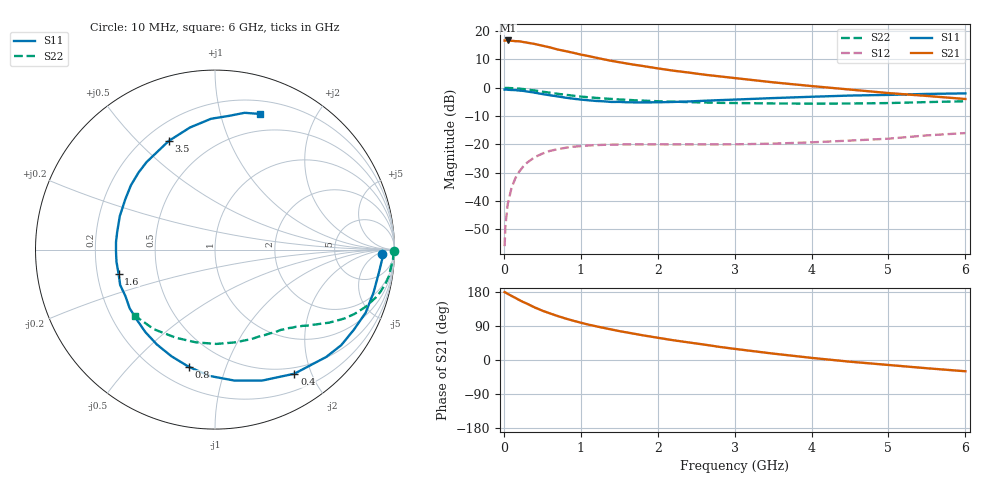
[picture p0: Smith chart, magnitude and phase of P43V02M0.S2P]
! SIEMENS Small Signal Semiconductors
! BFP182
! Si NPN RF Bipolar Junction Transistor in SOT143
! VCE = 3 V  IC = 2 mA
! Common Emitter S-Parameters:  March  1996
# GHz  S  MA  R  50
!  f  S11  S21  S12  S22
! GHz  MAG  ANG  MAG  ANG  MAG  ANG  MAG  ANG
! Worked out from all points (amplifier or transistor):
!   36 points, 10 MHz to 6 GHz, reference 50 ohm
!   highest |S21| = 16.7 dB at 50 MHz (marker M1)
!   |S21| within 3 dB of that: start of sweep to 673.9 MHz
!   unconditionally stable (mu >= 1): 2.189 GHz to 5.892 GHz
!   at 250 MHz: K = 0.13, MSG = 22.0 dB, |S12| = -27.9 dB
!   at 1.4 GHz: K = 0.68, MSG = 14.8 dB, |S12| = -20.1 dB
!   at 6 GHz: K = 0.99, MSG = 6.0 dB, |S12| = -16.0 dB
!   lowest NFmin = 1.10 dB at 450 MHz
!   S11 on the Smith chart (normalised r, x): 10 MHz: 24, -9; 400 MHz: 0.41, -1.75; 800 MHz: 0.32, -0.75; 1.6 GHz: 0.29, -0.11; 3.5 GHz: 0.29, +0.62; 6 GHz: 0.32, +1.34
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0.01  0.9298 -1.5  6.819 179.2  0.0016 85.0  0.9964 -0.5
0.02  0.9337 -3.0  6.823 178.4  0.0036 87.1  0.9934 -1.1
0.05  0.9226 -7.7  6.848 174.6  0.0088 87.6  0.9936 -2.9
0.1  0.9152 -15.0  6.75 169.2  0.0171 80.5  0.9852 -5.8
0.2  0.8929 -30.1  6.624 158.3  0.0331 72.4  0.968 -11.4
0.25  0.8822 -37.1  6.437 153.2  0.0405 68.5  0.952 -14.2
0.4  0.8208 -57.4  5.945 138.8  0.0595 57.6  0.8969 -20.9
0.5  0.7757 -70.1  5.534 130.2  0.0688 51.2  0.8555 -24.8
0.6  0.7375 -81.6  5.161 122.9  0.077 45.6  0.8185 -27.9
0.7  0.7048 -92.3  4.742 116.0  0.0824 41.0  0.7838 -30.4
0.8  0.6696 -102.5  4.445 109.6  0.0872 36.9  0.7539 -32.7
0.9  0.6419 -112.2  4.154 103.8  0.0912 33.3  0.7255 -34.6
1.1  0.6014 -130.2  3.631 93.3  0.0959 27.5  0.6805 -38.1
1.3  0.5771 -145.5  3.18 84.6  0.0985 23.2  0.6474 -41.0
1.6  0.5539 -166.0  2.678 72.7  0.1003 18.5  0.6135 -45.1
1.8  0.5517 -179.1  2.432 65.4  0.1002 16.8  0.5941 -47.7
2.2  0.5623 160.6  2.008 52.2  0.1003 13.9  0.5701 -53.6
2.8  0.6048 134.8  1.594 34.7  0.1003 13.2  0.5419 -63.7
3.5  0.6579 113.1  1.249 16.9  0.1033 14.3  0.529 -77.7
4.5  0.7294 91.7  0.93 -4.5  0.117 17.4  0.5276 -101.6
5.5  0.7798 77.8  0.718 -21.8  0.1445 17.9  0.559 -127.4
6  0.7965 71.5  0.634 -29.7  0.1587 14.8  0.578 -140.1
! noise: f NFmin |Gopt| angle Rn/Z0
0.45  1.1  0.42  29  0.36
0.9  1.2  0.4  58  0.3
1.8  1.85  0.32  126  0.22
